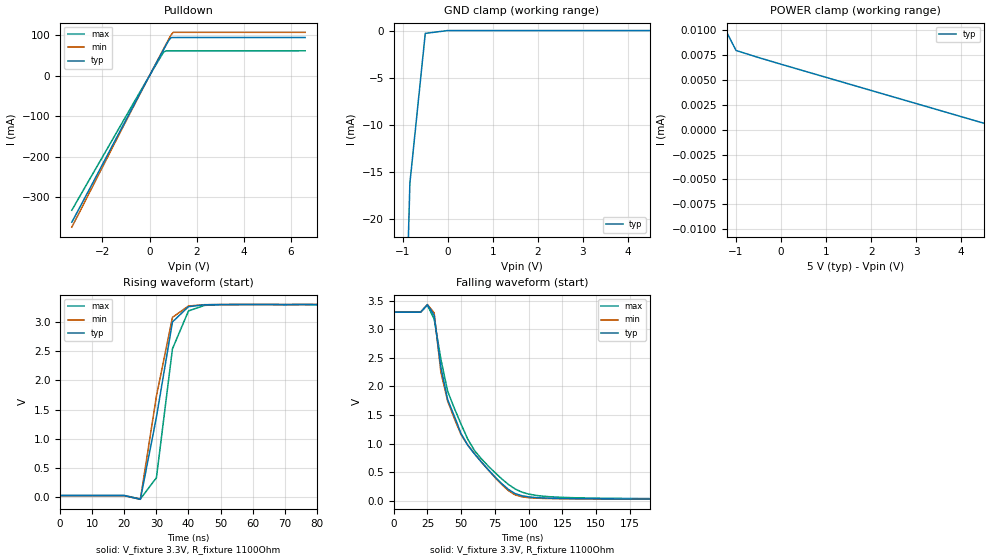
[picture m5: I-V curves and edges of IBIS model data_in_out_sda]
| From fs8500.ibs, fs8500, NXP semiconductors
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|   Model data_in_out_sda
[Model]   data_in_out_sda
Model_type   I/O_open_drain
Polarity   Non-Inverting
Vmeas = 1.65
Cref = 0pF
Rref = 1100Ohm
|   typ   min   max
C_comp   1.962p   1.78p   6.746p
Vinh  =   1.624
Vinl  =   1.383
[Model Spec]
Vmeas   1.65   1.5   1.8
Vref   3.3   3.1   3.5
|   typ min max
[Power Clamp Reference]  5.0 NA NA
[GND Clamp Reference]   0   NA NA
[pullup reference]   3.3 NA NA
[pulldown reference]   0   NA NA
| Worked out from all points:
|   slope of the pulldown table from 0 to 0.495 V, typ, clamps not added: 9.32 ohm
|   rising waveform, V_fixture 3.3V, R_fixture 1100Ohm: 20-80 % time 6.36ns typ, 6.36ns min, 5.01ns max; typ from 0.028 V to 3.3 V
|   falling waveform, V_fixture 3.3V, R_fixture 1100Ohm: 20-80 % time 31.6ns typ, 31.8ns min, 33.2ns max; typ from 3.3 V to 0.028 V
[GND Clamp]
|Voltage   I(typ)   I(min)   I(max)
-5V       -4A        NA         NA
-1.022V   -47.83mA   NA         NA
-838.4mV  -16.16mA   NA         NA
-497mV    -297.9uA   NA         NA
0V        0A         NA         NA
10V       5uA        NA         NA
[Power Clamp]
|Voltage   I(typ)   I(min)   I(max)
-5V       2A         NA         NA
-1.5V     12.36uA    NA         NA
-999.9mV  7.966uA    NA         NA
5V        0A         NA         NA
5.497V    -298.5uA   NA         NA
10V       -800uA     NA         NA
[Pulldown]
|Voltage   I(typ)   I(min)   I(max)
-3.3V     -360.7mA   -373mA     -331.4mA
-400mV    -43.42mA   -44.62mA   -39.73mA
600mV     64.26mA    66.27mA    58.04mA
800mV     85.27mA    88.1mA     60.66mA
900mV     93.19mA    98.91mA    60.7mA
1V        93.32mA    106.1mA    60.72mA
6.6V      93.38mA    106.2mA    60.81mA
|   typ   min   max
[Temperature Range]   27   -40   175
[Ramp]
R_load = 1100ohm
|   typ   min   max
dV/dt_r   308.1e-3/1e-9   307.1e-3/1e-9   316.3e-3/1e-9
dV/dt_f   56.59e-3/1e-9   52.35e-3/1e-9   57.28e-3/1e-9
[Rising Waveform]
V_fixture = 3.3V
R_fixture = 1100Ohm
|Time   V(typ)   V(min)   V(max)
0s        27.52mV    26.76mV    30.11mV
20ns      27.52mV    26.76mV    30.11mV
25ns      -36.06mV   -35.42mV   -30.17mV
30ns      1.37V      1.73V      332.8mV
35ns      3.001V     3.08V      2.541V
40ns      3.263V     3.274V     3.19V
45ns      3.295V     3.297V     3.285V
55ns      3.299V     3.3V       3.299V
490ns     3.3V       3.3V       3.3V
[Falling Waveform]
V_fixture = 3.3V
R_fixture = 1100Ohm
|Time   V(typ)   V(min)   V(max)
0s        3.3V       3.3V       3.3V
25ns      3.43V      3.434V     3.424V
30ns      3.248V     3.289V     3.181V
35ns      2.333V     2.249V     2.476V
40ns      1.77V      1.745V     1.917V
50ns      1.173V     1.153V     1.338V
60ns      817.5mV    821.9mV    875.6mV
90ns      126.4mV    104mV      207mV
140ns     37.51mV    33.61mV    51.26mV
490ns     27.67mV    26.81mV    31.07mV
